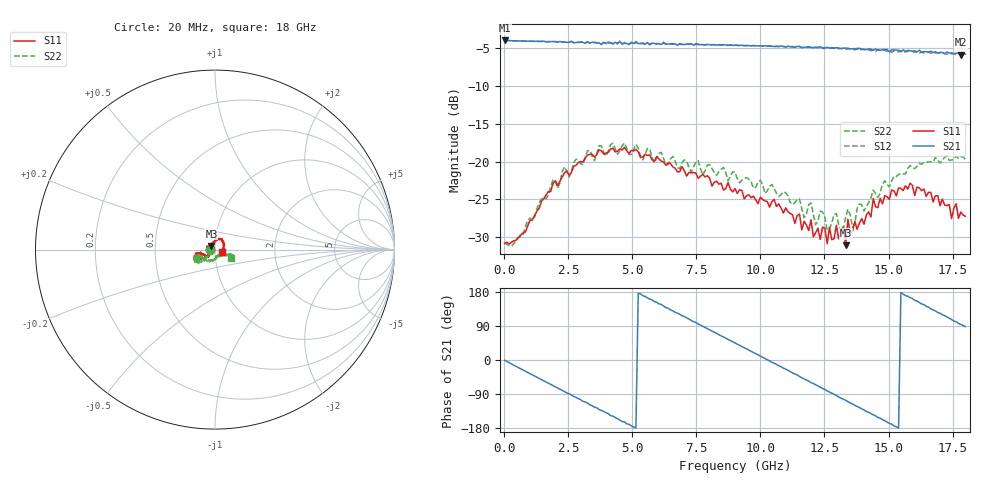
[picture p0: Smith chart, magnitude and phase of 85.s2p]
!Agilent Technologies,N5230A,US43500223,A.07.50.48
!Agilent N5230A: A.07.50.48
!Date: Wednesday, February 17, 2016 16:27:30
!Correction: S11(Full 2 Port(1,2))
!S21(Full 2 Port(1,2))
!S12(Full 2 Port(1,2))
!S22(Full 2 Port(1,2))
!S2P File: Measurements: S11, S21, S12, S22:
# Hz S  RI  R 50
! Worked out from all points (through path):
!   201 points, 20 MHz to 18 GHz, reference 50 ohm
!   highest |S21| = -3.98 dB at 20 MHz (marker M1); lowest = -5.9 dB at 17.82 GHz (marker M2)
!   group delay of S21, straight-line fit = 97.4 ps
!   lowest |S11| = -31.1 dB at 13.33 GHz (marker M3), VSWR 1.06, Z = 48 + j1.89 ohm
!   |S11| at or under -10 dB: start of sweep to end of sweep
!   |S22| runs from -31.2 to -17.5 dB; largest |S21 - S12| = 0.033
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2e7  -0.0288 0.000662  0.6321 -0.0084  0.6314 -0.00803  -0.029 0.000448
1.5483e9  -0.0443 -0.0356  0.3593 -0.5114  0.357 -0.5114  -0.0396 -0.0421
3.0766e9  -0.0836 -0.0528  -0.204 -0.579  -0.2012 -0.5817  -0.0787 -0.0541
4.515e9  -0.1112 -0.0489  -0.577 -0.2287  -0.5831 -0.2296  -0.1078 -0.0471
6.0433e9  -0.1014 -0.0235  -0.5114 0.318  -0.5051 0.3288  -0.1084 -0.0341
7.5716e9  -0.0751 -0.0194  -0.0518 0.5969  -0.0443 0.5917  -0.0875 -0.0515
9.01e9  -0.056 -0.0355  0.4155 0.4165  0.423 0.4072  -0.0587 -0.0611
1.03585e10  -0.0328 -0.0377  0.582 -0.0232  0.5782 -0.0353  -0.0298 -0.0617
1.15272e10  -0.0388 -0.0225  0.4175 -0.3973  0.4104 -0.407  -0.000494 -0.0566
1.1707e10  -0.0378 -0.0137  0.3693 -0.4359  0.3618 -0.4415  -0.00128 -0.0425
1.19767e10  -0.04 -0.0097  0.2856 -0.4919  0.2842 -0.4922  0.00448 -0.0531
1.20666e10  -0.0307 -0.00851  0.2665 -0.4995  0.2548 -0.511  0.00784 -0.044
1.32353e10  -0.0302 0.0211  -0.1323 -0.5462  -0.1494 -0.5368  0.0113 -0.034
1.33252e10  -0.0199 0.0196  -0.1576 -0.5406  -0.1737 -0.5238  0.0172 -0.0391
1.34151e10  -0.025 0.0331  -0.1921 -0.5275  -0.2044 -0.5175  0.0288 -0.039
1.35949e10  -0.0112 0.0326  -0.241 -0.5017  -0.2631 -0.4856  0.0261 -0.0258
1.38646e10  -0.0108 0.0377  -0.3264 -0.4576  -0.3375 -0.4302  0.0371 -0.037
1.4404e10  0.00219 0.057  -0.4425 -0.3168  -0.4554 -0.2993  0.0562 -0.0323
1.50333e10  0.0135 0.0546  -0.5182 -0.1195  -0.5299 -0.1004  0.0638 -0.0237
1.6202e10  0.0386 0.0548  -0.4814 0.2566  -0.4505 0.2664  0.0926 -0.0296
1.78202e10  0.0458 -0.00762  -0.0365 0.5076  -0.0119 0.5068  0.1014 -0.0363
1.8e10  0.0415 -0.0131  0.0168 0.5126  0.0421 0.5063  0.0914 -0.0484
